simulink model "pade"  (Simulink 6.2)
settings: Solver=ode45  StartTime=0.0  StopTime=5  MaxStep=0.05  RelTol=1e-3  AbsTol=1e-3
undefined symbols (not defined in the file or in its folder): T

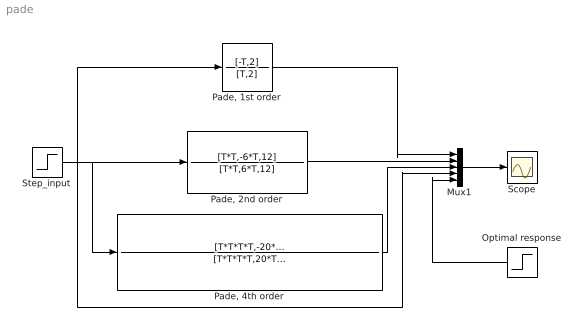
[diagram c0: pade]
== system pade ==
  Mux1 : Mux  Inputs=5
  Optimal response : Step  Orientation=left  Time=2  SampleTime=0
  "Pade, 1st order" : TransferFcn  Numerator=[-T,2]  Denominator=[T,2]
  "Pade, 2nd order" : TransferFcn  Numerator=[T*T,-6*T,12]  Denominator=[T*T,6*T,12]
  "Pade, 4th order" : TransferFcn  Numerator=[T*T*T*T,-20*T*T*T,180*T*T,-840*T,1680]  Denominator=[T*T*T*T,20*T*T*T,180*T*T,840*T,1680]
  Scope : Scope
  Step_input : Step  SampleTime=0
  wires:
  Step_input/1 -> "Pade, 1st order"/1, "Pade, 2nd order"/1, "Pade, 4th order"/1, Mux1/4
  "Pade, 1st order"/1 -> Mux1/1
  "Pade, 2nd order"/1 -> Mux1/2
  "Pade, 4th order"/1 -> Mux1/3
  Optimal response/1 -> Mux1/5
  Mux1/1 -> Scope/1
